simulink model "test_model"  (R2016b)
settings: Solver=VariableStepAuto  StartTime=0.0  StopTime=runtime  RelTol=1e-3
InitFcn:
  | clear mex
  | delete test_model_sfun.mexw64
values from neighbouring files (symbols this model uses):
  g = 9.81    [modelParameters.m]
  height_controlled_o = (((Rm*If        + (((omega0_o * 2 * Rm * Kv * Kq      * Kd + 1)^2) - 1)/(4* Rm*Kv^2*Kq      * Kd))/Vb)*(Pmax - Pmin) + Pmin)    [modelParameters.m]
  If = 0.3836    [modelParameters.m]
  Jreq = 4.2012e-05    [modelParameters.m]
  Jxx = 0.0130    (= 0.013)    [modelParameters.m]
  Jyy = 0.0140    (= 0.014)    [modelParameters.m]
  Jzz = 0.0285    [modelParameters.m]
  Kd = 1.4852e-07    [modelParameters.m]
  Ki_mahony = 0.001    [modelParameters.m]
  Kp_mahony = 0.4    [modelParameters.m]
  Kq = 96.3422    [modelParameters.m]
  Kt = 1.2007e-05    [modelParameters.m]
  Kv = 96.3422    [modelParameters.m]
  m = 1.216    [modelParameters.m]
  omega0_o = sqrt((m*g)/(4*Kt))    [modelParameters.m]
  omega1_o = sqrt((m*g)/(4*Kt))    [modelParameters.m]
  omega2_o = sqrt((m*g)/(4*Kt))    [modelParameters.m]
  omega3_o = sqrt((m*g)/(4*Kt))    [modelParameters.m]
  pitch_o = 0    [modelParameters.m]
  pitchrate_o = 0    [modelParameters.m]
  Pmax = 1    [modelParameters.m]
  Pmin = 0    [modelParameters.m]
  r_oc = [0; 0; 0]    [modelParameters.m]
  rhx = 0.16    [modelParameters.m]
  rhy = 0.16    [modelParameters.m]
  rhz = 0.03    [modelParameters.m]
  Rm = 0.235    [modelParameters.m]
  roll_o = 0    [modelParameters.m]
  rollrate_o = 0    [modelParameters.m]
  Tc = 0.04    [modelParameters.m]
  Tq = 0.005    [modelParameters.m]
  Vb = 11.4    [modelParameters.m]
  x_controlled_o = 0    [modelParameters.m]
  x_o = 0    [modelParameters.m]
  x_vel_o = 0    [modelParameters.m]
  y_controlled_o = 0    [modelParameters.m]
  y_o = 0    [modelParameters.m]
  y_vel_o = 0    [modelParameters.m]
  yaw_controlled_o = 0    [modelParameters.m]
  yaw_o = 0    [modelParameters.m]
  yawrate_o = 0    [modelParameters.m]
  z_o = 0    [modelParameters.m]
  z_vel_o = 0    [modelParameters.m]
undefined symbols (not defined in the file or in its folder): a, Ki, Kp, Ts
libraries: simulink x38, dsparch4 x3, vrlib x2
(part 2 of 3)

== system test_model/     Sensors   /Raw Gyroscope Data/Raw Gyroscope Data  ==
  From Workspace5 : FromWorkspace  VariableName=raw_gyro_data  SampleTime=Tq
  raw_gyro : Outport
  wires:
  From Workspace5/1 -> raw_gyro/1

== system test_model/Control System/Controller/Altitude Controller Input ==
  note: 1) Add Subsystem or Model blocks as valid variant choices. 2) You cannot connect blocks at this level. At simulation, connectivity is automatically determined, based on the active variant and port name matching.
  z_error_model : Inport
  Feedback : Subsystem  VariantControl=logAnalysisToggle==0
  z error : Subsystem  VariantControl=logAnalysisToggle==1
  z_error : Outport

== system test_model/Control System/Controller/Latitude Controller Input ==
  note: 1) Add Subsystem or Model blocks as valid variant choices. 2) You cannot connect blocks at this level. At simulation, connectivity is automatically determined, based on the active variant and port name matching.
  x_error_model : Inport
  Feedback : Subsystem  VariantControl=logAnalysisToggle==0
  x error : Subsystem  VariantControl=logAnalysisToggle==1
  x_error : Outport

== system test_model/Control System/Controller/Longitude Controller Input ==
  note: 1) Add Subsystem or Model blocks as valid variant choices. 2) You cannot connect blocks at this level. At simulation, connectivity is automatically determined, based on the active variant and port name matching.
  y_error_model : Inport
  Feedback : Subsystem  VariantControl=logAnalysisToggle==0
  y error : Subsystem  VariantControl=logAnalysisToggle==1
  y_error : Outport

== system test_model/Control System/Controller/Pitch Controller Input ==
  note: 1) Add Subsystem or Model blocks as valid variant choices. 2) You cannot connect blocks at this level. At simulation, connectivity is automatically determined, based on the active variant and port name matching.
  pitch_error_model : Inport
  Feedback : Subsystem  VariantControl=logAnalysisToggle==0
  pitch error : Subsystem  VariantControl=logAnalysisToggle==1
  pitch_error : Outport

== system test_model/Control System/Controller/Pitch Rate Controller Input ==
  note: 1) Add Subsystem or Model blocks as valid variant choices. 2) You cannot connect blocks at this level. At simulation, connectivity is automatically determined, based on the active variant and port name matching.
  pitchrate_error_model : Inport
  Feedback : Subsystem  VariantControl=logAnalysisToggle==0
  pitchrate error : Subsystem  VariantControl=logAnalysisToggle==1
  pitchrate_error : Outport

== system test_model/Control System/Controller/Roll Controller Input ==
  note: 1) Add Subsystem or Model blocks as valid variant choices. 2) You cannot connect blocks at this level. At simulation, connectivity is automatically determined, based on the active variant and port name matching.
  roll_error_model : Inport
  Feedback : Subsystem  VariantControl=logAnalysisToggle==0
  roll error : Subsystem  VariantControl=logAnalysisToggle==1
  roll_error : Outport

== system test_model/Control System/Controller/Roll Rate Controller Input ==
  note: 1) Add Subsystem or Model blocks as valid variant choices. 2) You cannot connect blocks at this level. At simulation, connectivity is automatically determined, based on the active variant and port name matching.
  rollrate_error_model : Inport
  Feedback : Subsystem  VariantControl=logAnalysisToggle==0
  rollrate error : Subsystem  VariantControl=logAnalysisToggle==1
  rollrate_error : Outport

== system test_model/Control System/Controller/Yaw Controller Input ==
  note: 1) Add Subsystem or Model blocks as valid variant choices. 2) You cannot connect blocks at this level. At simulation, connectivity is automatically determined, based on the active variant and port name matching.
  yaw_error_model : Inport
  Feedback : Subsystem  VariantControl=logAnalysisToggle==0
  yaw error : Subsystem  VariantControl=logAnalysisToggle==1
  yaw_error : Outport

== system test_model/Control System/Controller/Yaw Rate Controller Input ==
  note: 1) Add Subsystem or Model blocks as valid variant choices. 2) You cannot connect blocks at this level. At simulation, connectivity is automatically determined, based on the active variant and port name matching.
  yawrate_error_model : Inport
  Feedback : Subsystem  VariantControl=logAnalysisToggle==0
  yawrate error : Subsystem  VariantControl=logAnalysisToggle==1
  yawrate_error : Outport

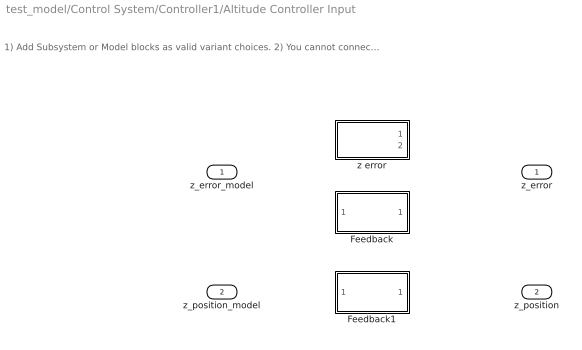
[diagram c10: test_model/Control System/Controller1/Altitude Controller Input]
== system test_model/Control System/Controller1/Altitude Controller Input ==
  note: 1) Add Subsystem or Model blocks as valid variant choices. 2) You cannot connect blocks at this level. At simulation, connectivity is automatically determined, based on the active variant and port name matching.
  z_error_model : Inport
  z_position_model : Inport  Port=2
  Feedback : Subsystem  VariantControl=logAnalysisToggle==0
  Feedback1 : Subsystem  VariantControl=logAnalysisToggle==0
  z error : Subsystem  VariantControl=logAnalysisToggle==1
  z_error : Outport
  z_position : Outport  Port=2

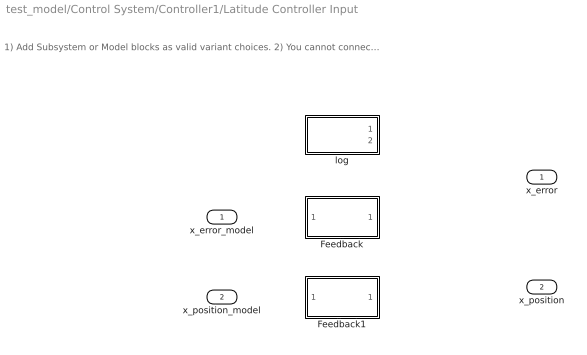
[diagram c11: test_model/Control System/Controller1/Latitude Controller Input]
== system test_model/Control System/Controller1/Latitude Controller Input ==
  note: 1) Add Subsystem or Model blocks as valid variant choices. 2) You cannot connect blocks at this level. At simulation, connectivity is automatically determined, based on the active variant and port name matching.
  x_error_model : Inport
  x_position_model : Inport  Port=2
  Feedback : Subsystem  VariantControl=logAnalysisToggle==0
  Feedback1 : Subsystem  VariantControl=logAnalysisToggle==0
  log : Subsystem  VariantControl=logAnalysisToggle==1
  x_error : Outport
  x_position : Outport  Port=2

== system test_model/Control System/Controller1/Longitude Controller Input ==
  note: 1) Add Subsystem or Model blocks as valid variant choices. 2) You cannot connect blocks at this level. At simulation, connectivity is automatically determined, based on the active variant and port name matching.
  y_error_model : Inport
  y_position_model : Inport  Port=2
  Feedback : Subsystem  VariantControl=logAnalysisToggle==0
  Feedback1 : Subsystem  VariantControl=logAnalysisToggle==0
  y error : Subsystem  VariantControl=logAnalysisToggle==1
  y_error : Outport
  y_position : Outport  Port=2

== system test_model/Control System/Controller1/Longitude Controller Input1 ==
  note: 1) Add Subsystem or Model blocks as valid variant choices. 2) You cannot connect blocks at this level. At simulation, connectivity is automatically determined, based on the active variant and port name matching.
  y_vel_error_model : Inport
  y_vel_model : Inport  Port=2
  Feedback : Subsystem  VariantControl=logAnalysisToggle==0
  Feedback1 : Subsystem  VariantControl=logAnalysisToggle==0
  y error : Subsystem  VariantControl=logAnalysisToggle==1
  y_vel_error : Outport
  y_vel : Outport  Port=2

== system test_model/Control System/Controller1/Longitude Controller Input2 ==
  note: 1) Add Subsystem or Model blocks as valid variant choices. 2) You cannot connect blocks at this level. At simulation, connectivity is automatically determined, based on the active variant and port name matching.
  x_vel_error_model : Inport
  x_vel_model : Inport  Port=2
  Feedback : Subsystem  VariantControl=logAnalysisToggle==0
  Feedback1 : Subsystem  VariantControl=logAnalysisToggle==0
  y error : Subsystem  VariantControl=logAnalysisToggle==1
  x_vel_error : Outport
  x_vel : Outport  Port=2

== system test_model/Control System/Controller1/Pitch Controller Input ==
  note: 1) Add Subsystem or Model blocks as valid variant choices. 2) You cannot connect blocks at this level. At simulation, connectivity is automatically determined, based on the active variant and port name matching.
  pitch_error_model : Inport
  pitch_angle_model : Inport  Port=2
  Feedback : Subsystem  VariantControl=logAnalysisToggle==0
  Feedback1 : Subsystem  VariantControl=logAnalysisToggle==0
  pitch error : Subsystem  VariantControl=logAnalysisToggle==1
  pitch_error : Outport
  pitch_angle : Outport  Port=2

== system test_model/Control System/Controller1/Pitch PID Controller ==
  pitch_error : Inport
  pitch_angle : Inport  Port=2
  Add : Sum  Inputs=+-
  Discrete D Controller : Subsystem  TreatAsAtomicUnit=on  SystemSampleTime=Ts
  Discrete PI Controller : simulink/Continuous/PID Controller  Controller=PI  TimeDomain=Discrete-time  SampleTime=Ts  IntegratorMethod=Forward Euler  FilterMethod=Forward Euler  Form=Parallel  UseFilter=on  ControllerParametersSource=internal  P=Kp  I=Ki  D=0  N=100  InitialConditionSource=internal  InitialConditionForIntegrator=0  InitialConditionForFilter=0  ExternalReset=none  LimitOutput=off  UpperSaturationLimit=inf  LowerSaturationLimit=-inf  LinearizeAsGain=off  AntiWindupMode=none  Kb=1  TrackingMode=off  Kt=1  PParamMin=[]  PParamMax=[]  IParamMin=[]  IParamMax=[]  DParamMin=[]  DParamMax=[]  NParamMin=[]  NParamMax=[]  KbParamMin=[]  KbParamMax=[]  KtParamMin=[]  KtParamMax=[]  POutMin=[]  POutMax=[]  IOutMin=[]  IOutMax=[]  DOutMin=[]  DOutMax=[]  NOutMin=[]  NOutMax=[]  KbOutMin=[]  KbOutMax=[]  KtOutMin=[]  KtOutMax=[]  IntegratorOutMin=[]  IntegratorOutMax=[]  FilterOutMin=[]  FilterOutMax=[]  SumOutMin=[]  SumOutMax=[]  SumI1OutMin=[]  SumI1OutMax=[]  SumI2OutMin=[]  SumI2OutMax=[]  SumI3OutMin=[]  SumI3OutMax=[]  SumDOutMin=[]  SumDOutMax=[]  SaturationOutMin=[]  SaturationOutMax=[]  IntegratorContinuousStateAttributes=''  IntegratorStateMustResolveToSignalObject=off  IntegratorRTWStateStorageClass=Auto  FilterContinuousStateAttributes=''  FilterStateMustResolveToSignalObject=off  FilterRTWStateStorageClass=Auto  DifferentiatorICPrevScaledInput=0  DifferentiatorOutMin=[]  DifferentiatorOutMax=[]
  pitchrate_setpoint : Outport
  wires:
  pitch_angle/1 -> Discrete D Controller/1(pitch_angle)
  pitch_error/1 -> Discrete PI Controller/1
  Discrete PI Controller/1 -> Add/1
  Discrete D Controller/1(output) -> Add/2
  Add/1 -> pitchrate_setpoint/1

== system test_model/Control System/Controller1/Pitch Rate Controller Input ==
  note: 1) Add Subsystem or Model blocks as valid variant choices. 2) You cannot connect blocks at this level. At simulation, connectivity is automatically determined, based on the active variant and port name matching.
  pitchrate_error_model : Inport
  pitchrate_model : Inport  Port=2
  Feedback : Subsystem  VariantControl=logAnalysisToggle==0
  Feedback1 : Subsystem  VariantControl=logAnalysisToggle==0
  pitchrate error : Subsystem  VariantControl=logAnalysisToggle==1
  pitchrate_error : Outport
  pitchrate : Outport  Port=2

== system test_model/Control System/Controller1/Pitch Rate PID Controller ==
  pitchrate_error : Inport
  pitchrate : Inport  Port=2
  Add : Sum  Inputs=+-
  Discrete D Controller : Subsystem  TreatAsAtomicUnit=on  SystemSampleTime=Ts
  Discrete PI Controller : simulink/Continuous/PID Controller  Controller=PI  TimeDomain=Discrete-time  SampleTime=Ts  IntegratorMethod=Forward Euler  FilterMethod=Forward Euler  Form=Parallel  UseFilter=on  ControllerParametersSource=internal  P=Kp  I=Ki  D=0  N=100  InitialConditionSource=internal  InitialConditionForIntegrator=0  InitialConditionForFilter=0  ExternalReset=none  LimitOutput=off  UpperSaturationLimit=inf  LowerSaturationLimit=-inf  LinearizeAsGain=off  AntiWindupMode=none  Kb=1  TrackingMode=off  Kt=1  PParamMin=[]  PParamMax=[]  IParamMin=[]  IParamMax=[]  DParamMin=[]  DParamMax=[]  NParamMin=[]  NParamMax=[]  KbParamMin=[]  KbParamMax=[]  KtParamMin=[]  KtParamMax=[]  POutMin=[]  POutMax=[]  IOutMin=[]  IOutMax=[]  DOutMin=[]  DOutMax=[]  NOutMin=[]  NOutMax=[]  KbOutMin=[]  KbOutMax=[]  KtOutMin=[]  KtOutMax=[]  IntegratorOutMin=[]  IntegratorOutMax=[]  FilterOutMin=[]  FilterOutMax=[]  SumOutMin=[]  SumOutMax=[]  SumI1OutMin=[]  SumI1OutMax=[]  SumI2OutMin=[]  SumI2OutMax=[]  SumI3OutMin=[]  SumI3OutMax=[]  SumDOutMin=[]  SumDOutMax=[]  SaturationOutMin=[]  SaturationOutMax=[]  IntegratorContinuousStateAttributes=''  IntegratorStateMustResolveToSignalObject=off  IntegratorRTWStateStorageClass=Auto  FilterContinuousStateAttributes=''  FilterStateMustResolveToSignalObject=off  FilterRTWStateStorageClass=Auto  DifferentiatorICPrevScaledInput=0  DifferentiatorOutMin=[]  DifferentiatorOutMax=[]
  x_motor_command : Outport
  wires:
  pitchrate/1 -> Discrete D Controller/1(pitch_angle)
  pitchrate_error/1 -> Discrete PI Controller/1
  Discrete PI Controller/1 -> Add/1
  Discrete D Controller/1(output) -> Add/2
  Add/1 -> x_motor_command/1

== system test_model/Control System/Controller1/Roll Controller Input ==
  note: 1) Add Subsystem or Model blocks as valid variant choices. 2) You cannot connect blocks at this level. At simulation, connectivity is automatically determined, based on the active variant and port name matching.
  roll_error_model : Inport
  roll_angle_model : Inport  Port=2
  Feedback : Subsystem  VariantControl=logAnalysisToggle==0
  Feedback1 : Subsystem  VariantControl=logAnalysisToggle==0
  roll error : Subsystem  VariantControl=logAnalysisToggle==1
  roll_error : Outport
  roll_angle : Outport  Port=2

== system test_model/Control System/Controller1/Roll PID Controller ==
  roll_error : Inport
  roll_angle : Inport  Port=2
  Add : Sum  Inputs=+-
  Discrete D Controller : Subsystem  TreatAsAtomicUnit=on  SystemSampleTime=Ts
  Discrete PI Controller : simulink/Continuous/PID Controller  Controller=PI  TimeDomain=Discrete-time  SampleTime=Ts  IntegratorMethod=Forward Euler  FilterMethod=Forward Euler  Form=Parallel  UseFilter=on  ControllerParametersSource=internal  P=Kp  I=Ki  D=0  N=100  InitialConditionSource=internal  InitialConditionForIntegrator=0  InitialConditionForFilter=0  ExternalReset=none  LimitOutput=off  UpperSaturationLimit=inf  LowerSaturationLimit=-inf  LinearizeAsGain=off  AntiWindupMode=none  Kb=1  TrackingMode=off  Kt=1  PParamMin=[]  PParamMax=[]  IParamMin=[]  IParamMax=[]  DParamMin=[]  DParamMax=[]  NParamMin=[]  NParamMax=[]  KbParamMin=[]  KbParamMax=[]  KtParamMin=[]  KtParamMax=[]  POutMin=[]  POutMax=[]  IOutMin=[]  IOutMax=[]  DOutMin=[]  DOutMax=[]  NOutMin=[]  NOutMax=[]  KbOutMin=[]  KbOutMax=[]  KtOutMin=[]  KtOutMax=[]  IntegratorOutMin=[]  IntegratorOutMax=[]  FilterOutMin=[]  FilterOutMax=[]  SumOutMin=[]  SumOutMax=[]  SumI1OutMin=[]  SumI1OutMax=[]  SumI2OutMin=[]  SumI2OutMax=[]  SumI3OutMin=[]  SumI3OutMax=[]  SumDOutMin=[]  SumDOutMax=[]  SaturationOutMin=[]  SaturationOutMax=[]  IntegratorContinuousStateAttributes=''  IntegratorStateMustResolveToSignalObject=off  IntegratorRTWStateStorageClass=Auto  FilterContinuousStateAttributes=''  FilterStateMustResolveToSignalObject=off  FilterRTWStateStorageClass=Auto  DifferentiatorICPrevScaledInput=0  DifferentiatorOutMin=[]  DifferentiatorOutMax=[]
  rollrate_setpoint : Outport
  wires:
  roll_angle/1 -> Discrete D Controller/1(pitch_angle)
  roll_error/1 -> Discrete PI Controller/1
  Discrete PI Controller/1 -> Add/1
  Discrete D Controller/1(output) -> Add/2
  Add/1 -> rollrate_setpoint/1

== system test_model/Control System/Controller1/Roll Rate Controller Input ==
  note: 1) Add Subsystem or Model blocks as valid variant choices. 2) You cannot connect blocks at this level. At simulation, connectivity is automatically determined, based on the active variant and port name matching.
  rollrate_error_model : Inport
  rollrate_model : Inport  Port=2
  Feedback : Subsystem  VariantControl=logAnalysisToggle==0
  Feedback1 : Subsystem  VariantControl=logAnalysisToggle==0
  rollrate error : Subsystem  VariantControl=logAnalysisToggle==1
  rollrate_error : Outport
  rollrate : Outport  Port=2

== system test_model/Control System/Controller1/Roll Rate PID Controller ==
  rollrate_error : Inport
  rollrate : Inport  Port=2
  Add : Sum  Inputs=+-
  Discrete D Controller : Subsystem  TreatAsAtomicUnit=on  SystemSampleTime=Ts
  Discrete PI Controller : simulink/Continuous/PID Controller  Controller=PI  TimeDomain=Discrete-time  SampleTime=Ts  IntegratorMethod=Forward Euler  FilterMethod=Forward Euler  Form=Parallel  UseFilter=on  ControllerParametersSource=internal  P=Kp  I=Ki  D=0  N=100  InitialConditionSource=internal  InitialConditionForIntegrator=0  InitialConditionForFilter=0  ExternalReset=none  LimitOutput=off  UpperSaturationLimit=inf  LowerSaturationLimit=-inf  LinearizeAsGain=off  AntiWindupMode=none  Kb=1  TrackingMode=off  Kt=1  PParamMin=[]  PParamMax=[]  IParamMin=[]  IParamMax=[]  DParamMin=[]  DParamMax=[]  NParamMin=[]  NParamMax=[]  KbParamMin=[]  KbParamMax=[]  KtParamMin=[]  KtParamMax=[]  POutMin=[]  POutMax=[]  IOutMin=[]  IOutMax=[]  DOutMin=[]  DOutMax=[]  NOutMin=[]  NOutMax=[]  KbOutMin=[]  KbOutMax=[]  KtOutMin=[]  KtOutMax=[]  IntegratorOutMin=[]  IntegratorOutMax=[]  FilterOutMin=[]  FilterOutMax=[]  SumOutMin=[]  SumOutMax=[]  SumI1OutMin=[]  SumI1OutMax=[]  SumI2OutMin=[]  SumI2OutMax=[]  SumI3OutMin=[]  SumI3OutMax=[]  SumDOutMin=[]  SumDOutMax=[]  SaturationOutMin=[]  SaturationOutMax=[]  IntegratorContinuousStateAttributes=''  IntegratorStateMustResolveToSignalObject=off  IntegratorRTWStateStorageClass=Auto  FilterContinuousStateAttributes=''  FilterStateMustResolveToSignalObject=off  FilterRTWStateStorageClass=Auto  DifferentiatorICPrevScaledInput=0  DifferentiatorOutMin=[]  DifferentiatorOutMax=[]
  y_motor_command : Outport
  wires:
  rollrate/1 -> Discrete D Controller/1(pitch_angle)
  rollrate_error/1 -> Discrete PI Controller/1
  Discrete PI Controller/1 -> Add/1
  Discrete D Controller/1(output) -> Add/2
  Add/1 -> y_motor_command/1

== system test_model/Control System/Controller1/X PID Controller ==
  x_error : Inport
  x_pos : Inport  Port=2
  Add : Sum  Inputs=+-
  Discrete D Controller : Subsystem  TreatAsAtomicUnit=on  SystemSampleTime=Ts
  Discrete PI Controller : simulink/Continuous/PID Controller  Controller=PI  TimeDomain=Discrete-time  SampleTime=Ts  IntegratorMethod=Forward Euler  FilterMethod=Forward Euler  Form=Parallel  UseFilter=on  ControllerParametersSource=internal  P=Kp  I=Ki  D=0  N=100  InitialConditionSource=internal  InitialConditionForIntegrator=0  InitialConditionForFilter=0  ExternalReset=none  LimitOutput=off  UpperSaturationLimit=inf  LowerSaturationLimit=-inf  LinearizeAsGain=off  AntiWindupMode=none  Kb=1  TrackingMode=off  Kt=1  PParamMin=[]  PParamMax=[]  IParamMin=[]  IParamMax=[]  DParamMin=[]  DParamMax=[]  NParamMin=[]  NParamMax=[]  KbParamMin=[]  KbParamMax=[]  KtParamMin=[]  KtParamMax=[]  POutMin=[]  POutMax=[]  IOutMin=[]  IOutMax=[]  DOutMin=[]  DOutMax=[]  NOutMin=[]  NOutMax=[]  KbOutMin=[]  KbOutMax=[]  KtOutMin=[]  KtOutMax=[]  IntegratorOutMin=[]  IntegratorOutMax=[]  FilterOutMin=[]  FilterOutMax=[]  SumOutMin=[]  SumOutMax=[]  SumI1OutMin=[]  SumI1OutMax=[]  SumI2OutMin=[]  SumI2OutMax=[]  SumI3OutMin=[]  SumI3OutMax=[]  SumDOutMin=[]  SumDOutMax=[]  SaturationOutMin=[]  SaturationOutMax=[]  IntegratorContinuousStateAttributes=''  IntegratorStateMustResolveToSignalObject=off  IntegratorRTWStateStorageClass=Auto  FilterContinuousStateAttributes=''  FilterStateMustResolveToSignalObject=off  FilterRTWStateStorageClass=Auto  DifferentiatorICPrevScaledInput=0  DifferentiatorOutMin=[]  DifferentiatorOutMax=[]
  pitch_setpoint : Outport
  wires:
  x_pos/1 -> Discrete D Controller/1(x_pos)
  x_error/1 -> Discrete PI Controller/1
  Discrete PI Controller/1 -> Add/1
  Discrete D Controller/1(output) -> Add/2
  Add/1 -> pitch_setpoint/1

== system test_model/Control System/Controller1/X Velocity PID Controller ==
  x_vel_error : Inport
  x_vel : Inport  Port=2
  Add : Sum  Inputs=+-
  Discrete D Controller : Subsystem  TreatAsAtomicUnit=on  SystemSampleTime=Ts
  Discrete PI Controller : simulink/Continuous/PID Controller  Controller=PI  TimeDomain=Discrete-time  SampleTime=Ts  IntegratorMethod=Forward Euler  FilterMethod=Forward Euler  Form=Parallel  UseFilter=on  ControllerParametersSource=internal  P=Kp  I=Ki  D=0  N=100  InitialConditionSource=internal  InitialConditionForIntegrator=0  InitialConditionForFilter=0  ExternalReset=none  LimitOutput=off  UpperSaturationLimit=inf  LowerSaturationLimit=-inf  LinearizeAsGain=off  AntiWindupMode=none  Kb=1  TrackingMode=off  Kt=1  PParamMin=[]  PParamMax=[]  IParamMin=[]  IParamMax=[]  DParamMin=[]  DParamMax=[]  NParamMin=[]  NParamMax=[]  KbParamMin=[]  KbParamMax=[]  KtParamMin=[]  KtParamMax=[]  POutMin=[]  POutMax=[]  IOutMin=[]  IOutMax=[]  DOutMin=[]  DOutMax=[]  NOutMin=[]  NOutMax=[]  KbOutMin=[]  KbOutMax=[]  KtOutMin=[]  KtOutMax=[]  IntegratorOutMin=[]  IntegratorOutMax=[]  FilterOutMin=[]  FilterOutMax=[]  SumOutMin=[]  SumOutMax=[]  SumI1OutMin=[]  SumI1OutMax=[]  SumI2OutMin=[]  SumI2OutMax=[]  SumI3OutMin=[]  SumI3OutMax=[]  SumDOutMin=[]  SumDOutMax=[]  SaturationOutMin=[]  SaturationOutMax=[]  IntegratorContinuousStateAttributes=''  IntegratorStateMustResolveToSignalObject=off  IntegratorRTWStateStorageClass=Auto  FilterContinuousStateAttributes=''  FilterStateMustResolveToSignalObject=off  FilterRTWStateStorageClass=Auto  DifferentiatorICPrevScaledInput=0  DifferentiatorOutMin=[]  DifferentiatorOutMax=[]
  pitch_setpoint : Outport
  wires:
  x_vel/1 -> Discrete D Controller/1(x_vel)
  x_vel_error/1 -> Discrete PI Controller/1
  Discrete PI Controller/1 -> Add/1
  Discrete D Controller/1(output) -> Add/2
  Add/1 -> pitch_setpoint/1

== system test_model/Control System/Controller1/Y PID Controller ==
  y_error : Inport
  y_pos : Inport  Port=2
  Add : Sum  Inputs=+-
  Discrete D Controller : Subsystem  TreatAsAtomicUnit=on  SystemSampleTime=Ts
  Discrete PI Controller : simulink/Continuous/PID Controller  Controller=PI  TimeDomain=Discrete-time  SampleTime=Ts  IntegratorMethod=Forward Euler  FilterMethod=Forward Euler  Form=Parallel  UseFilter=on  ControllerParametersSource=internal  P=Kp  I=Ki  D=0  N=100  InitialConditionSource=internal  InitialConditionForIntegrator=0  InitialConditionForFilter=0  ExternalReset=none  LimitOutput=off  UpperSaturationLimit=inf  LowerSaturationLimit=-inf  LinearizeAsGain=off  AntiWindupMode=none  Kb=1  TrackingMode=off  Kt=1  PParamMin=[]  PParamMax=[]  IParamMin=[]  IParamMax=[]  DParamMin=[]  DParamMax=[]  NParamMin=[]  NParamMax=[]  KbParamMin=[]  KbParamMax=[]  KtParamMin=[]  KtParamMax=[]  POutMin=[]  POutMax=[]  IOutMin=[]  IOutMax=[]  DOutMin=[]  DOutMax=[]  NOutMin=[]  NOutMax=[]  KbOutMin=[]  KbOutMax=[]  KtOutMin=[]  KtOutMax=[]  IntegratorOutMin=[]  IntegratorOutMax=[]  FilterOutMin=[]  FilterOutMax=[]  SumOutMin=[]  SumOutMax=[]  SumI1OutMin=[]  SumI1OutMax=[]  SumI2OutMin=[]  SumI2OutMax=[]  SumI3OutMin=[]  SumI3OutMax=[]  SumDOutMin=[]  SumDOutMax=[]  SaturationOutMin=[]  SaturationOutMax=[]  IntegratorContinuousStateAttributes=''  IntegratorStateMustResolveToSignalObject=off  IntegratorRTWStateStorageClass=Auto  FilterContinuousStateAttributes=''  FilterStateMustResolveToSignalObject=off  FilterRTWStateStorageClass=Auto  DifferentiatorICPrevScaledInput=0  DifferentiatorOutMin=[]  DifferentiatorOutMax=[]
  roll_setpoint : Outport
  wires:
  y_pos/1 -> Discrete D Controller/1(y_pos)
  y_error/1 -> Discrete PI Controller/1
  Discrete PI Controller/1 -> Add/1
  Discrete D Controller/1(output) -> Add/2
  Add/1 -> roll_setpoint/1

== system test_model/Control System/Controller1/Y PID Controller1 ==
  y_error : Inport
  y_pos : Inport  Port=2
  Add : Sum  Inputs=+-
  Discrete D Controller : Subsystem  TreatAsAtomicUnit=on  SystemSampleTime=Ts
  Discrete PI Controller : simulink/Continuous/PID Controller  Controller=PI  TimeDomain=Discrete-time  SampleTime=Ts  IntegratorMethod=Forward Euler  FilterMethod=Forward Euler  Form=Parallel  UseFilter=on  ControllerParametersSource=internal  P=Kp  I=Ki  D=0  N=100  InitialConditionSource=internal  InitialConditionForIntegrator=0  InitialConditionForFilter=0  ExternalReset=none  LimitOutput=off  UpperSaturationLimit=inf  LowerSaturationLimit=-inf  LinearizeAsGain=off  AntiWindupMode=none  Kb=1  TrackingMode=off  Kt=1  PParamMin=[]  PParamMax=[]  IParamMin=[]  IParamMax=[]  DParamMin=[]  DParamMax=[]  NParamMin=[]  NParamMax=[]  KbParamMin=[]  KbParamMax=[]  KtParamMin=[]  KtParamMax=[]  POutMin=[]  POutMax=[]  IOutMin=[]  IOutMax=[]  DOutMin=[]  DOutMax=[]  NOutMin=[]  NOutMax=[]  KbOutMin=[]  KbOutMax=[]  KtOutMin=[]  KtOutMax=[]  IntegratorOutMin=[]  IntegratorOutMax=[]  FilterOutMin=[]  FilterOutMax=[]  SumOutMin=[]  SumOutMax=[]  SumI1OutMin=[]  SumI1OutMax=[]  SumI2OutMin=[]  SumI2OutMax=[]  SumI3OutMin=[]  SumI3OutMax=[]  SumDOutMin=[]  SumDOutMax=[]  SaturationOutMin=[]  SaturationOutMax=[]  IntegratorContinuousStateAttributes=''  IntegratorStateMustResolveToSignalObject=off  IntegratorRTWStateStorageClass=Auto  FilterContinuousStateAttributes=''  FilterStateMustResolveToSignalObject=off  FilterRTWStateStorageClass=Auto  DifferentiatorICPrevScaledInput=0  DifferentiatorOutMin=[]  DifferentiatorOutMax=[]
  y_vel_setpoint : Outport
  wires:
  y_pos/1 -> Discrete D Controller/1(y_pos)
  y_error/1 -> Discrete PI Controller/1
  Discrete PI Controller/1 -> Add/1
  Discrete D Controller/1(output) -> Add/2
  Add/1 -> y_vel_setpoint/1

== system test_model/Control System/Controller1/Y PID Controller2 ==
  x_error : Inport
  x_pos : Inport  Port=2
  Add : Sum  Inputs=+-
  Discrete D Controller : Subsystem  TreatAsAtomicUnit=on  SystemSampleTime=Ts
  Discrete PI Controller : simulink/Continuous/PID Controller  Controller=PI  TimeDomain=Discrete-time  SampleTime=Ts  IntegratorMethod=Forward Euler  FilterMethod=Forward Euler  Form=Parallel  UseFilter=on  ControllerParametersSource=internal  P=Kp  I=Ki  D=0  N=100  InitialConditionSource=internal  InitialConditionForIntegrator=0  InitialConditionForFilter=0  ExternalReset=none  LimitOutput=off  UpperSaturationLimit=inf  LowerSaturationLimit=-inf  LinearizeAsGain=off  AntiWindupMode=none  Kb=1  TrackingMode=off  Kt=1  PParamMin=[]  PParamMax=[]  IParamMin=[]  IParamMax=[]  DParamMin=[]  DParamMax=[]  NParamMin=[]  NParamMax=[]  KbParamMin=[]  KbParamMax=[]  KtParamMin=[]  KtParamMax=[]  POutMin=[]  POutMax=[]  IOutMin=[]  IOutMax=[]  DOutMin=[]  DOutMax=[]  NOutMin=[]  NOutMax=[]  KbOutMin=[]  KbOutMax=[]  KtOutMin=[]  KtOutMax=[]  IntegratorOutMin=[]  IntegratorOutMax=[]  FilterOutMin=[]  FilterOutMax=[]  SumOutMin=[]  SumOutMax=[]  SumI1OutMin=[]  SumI1OutMax=[]  SumI2OutMin=[]  SumI2OutMax=[]  SumI3OutMin=[]  SumI3OutMax=[]  SumDOutMin=[]  SumDOutMax=[]  SaturationOutMin=[]  SaturationOutMax=[]  IntegratorContinuousStateAttributes=''  IntegratorStateMustResolveToSignalObject=off  IntegratorRTWStateStorageClass=Auto  FilterContinuousStateAttributes=''  FilterStateMustResolveToSignalObject=off  FilterRTWStateStorageClass=Auto  DifferentiatorICPrevScaledInput=0  DifferentiatorOutMin=[]  DifferentiatorOutMax=[]
  x_vel_setpoint : Outport
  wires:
  x_pos/1 -> Discrete D Controller/1(x_pos)
  x_error/1 -> Discrete PI Controller/1
  Discrete PI Controller/1 -> Add/1
  Discrete D Controller/1(output) -> Add/2
  Add/1 -> x_vel_setpoint/1

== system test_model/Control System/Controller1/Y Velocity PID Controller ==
  y_error : Inport
  y_pos : Inport  Port=2
  Add : Sum  Inputs=+-
  Discrete D Controller : Subsystem  TreatAsAtomicUnit=on  SystemSampleTime=Ts
  Discrete PI Controller : simulink/Continuous/PID Controller  Controller=PI  TimeDomain=Discrete-time  SampleTime=Ts  IntegratorMethod=Forward Euler  FilterMethod=Forward Euler  Form=Parallel  UseFilter=on  ControllerParametersSource=internal  P=Kp  I=Ki  D=0  N=100  InitialConditionSource=internal  InitialConditionForIntegrator=0  InitialConditionForFilter=0  ExternalReset=none  LimitOutput=off  UpperSaturationLimit=inf  LowerSaturationLimit=-inf  LinearizeAsGain=off  AntiWindupMode=none  Kb=1  TrackingMode=off  Kt=1  PParamMin=[]  PParamMax=[]  IParamMin=[]  IParamMax=[]  DParamMin=[]  DParamMax=[]  NParamMin=[]  NParamMax=[]  KbParamMin=[]  KbParamMax=[]  KtParamMin=[]  KtParamMax=[]  POutMin=[]  POutMax=[]  IOutMin=[]  IOutMax=[]  DOutMin=[]  DOutMax=[]  NOutMin=[]  NOutMax=[]  KbOutMin=[]  KbOutMax=[]  KtOutMin=[]  KtOutMax=[]  IntegratorOutMin=[]  IntegratorOutMax=[]  FilterOutMin=[]  FilterOutMax=[]  SumOutMin=[]  SumOutMax=[]  SumI1OutMin=[]  SumI1OutMax=[]  SumI2OutMin=[]  SumI2OutMax=[]  SumI3OutMin=[]  SumI3OutMax=[]  SumDOutMin=[]  SumDOutMax=[]  SaturationOutMin=[]  SaturationOutMax=[]  IntegratorContinuousStateAttributes=''  IntegratorStateMustResolveToSignalObject=off  IntegratorRTWStateStorageClass=Auto  FilterContinuousStateAttributes=''  FilterStateMustResolveToSignalObject=off  FilterRTWStateStorageClass=Auto  DifferentiatorICPrevScaledInput=0  DifferentiatorOutMin=[]  DifferentiatorOutMax=[]
  roll_setpoint : Outport
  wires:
  y_pos/1 -> Discrete D Controller/1(y_pos)
  y_error/1 -> Discrete PI Controller/1
  Discrete PI Controller/1 -> Add/1
  Discrete D Controller/1(output) -> Add/2
  Add/1 -> roll_setpoint/1

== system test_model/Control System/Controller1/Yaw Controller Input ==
  note: 1) Add Subsystem or Model blocks as valid variant choices. 2) You cannot connect blocks at this level. At simulation, connectivity is automatically determined, based on the active variant and port name matching.
  yaw_error_model : Inport
  yaw_angle_model : Inport  Port=2
  Feedback : Subsystem  VariantControl=logAnalysisToggle==0
  Feedback1 : Subsystem  VariantControl=logAnalysisToggle==0
  yaw error : Subsystem  VariantControl=logAnalysisToggle==1
  yaw_error : Outport
  yaw_angle : Outport  Port=2

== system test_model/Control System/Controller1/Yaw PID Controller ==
  yaw_error : Inport
  yaw_angle : Inport  Port=2
  Add : Sum  Inputs=+-
  Discrete D Controller : Subsystem  TreatAsAtomicUnit=on  SystemSampleTime=Ts
  Discrete PI Controller : simulink/Continuous/PID Controller  Controller=PI  TimeDomain=Discrete-time  SampleTime=Ts  IntegratorMethod=Forward Euler  FilterMethod=Forward Euler  Form=Parallel  UseFilter=on  ControllerParametersSource=internal  P=Kp  I=Ki  D=0  N=100  InitialConditionSource=internal  InitialConditionForIntegrator=0  InitialConditionForFilter=0  ExternalReset=none  LimitOutput=off  UpperSaturationLimit=inf  LowerSaturationLimit=-inf  LinearizeAsGain=off  AntiWindupMode=none  Kb=1  TrackingMode=off  Kt=1  PParamMin=[]  PParamMax=[]  IParamMin=[]  IParamMax=[]  DParamMin=[]  DParamMax=[]  NParamMin=[]  NParamMax=[]  KbParamMin=[]  KbParamMax=[]  KtParamMin=[]  KtParamMax=[]  POutMin=[]  POutMax=[]  IOutMin=[]  IOutMax=[]  DOutMin=[]  DOutMax=[]  NOutMin=[]  NOutMax=[]  KbOutMin=[]  KbOutMax=[]  KtOutMin=[]  KtOutMax=[]  IntegratorOutMin=[]  IntegratorOutMax=[]  FilterOutMin=[]  FilterOutMax=[]  SumOutMin=[]  SumOutMax=[]  SumI1OutMin=[]  SumI1OutMax=[]  SumI2OutMin=[]  SumI2OutMax=[]  SumI3OutMin=[]  SumI3OutMax=[]  SumDOutMin=[]  SumDOutMax=[]  SaturationOutMin=[]  SaturationOutMax=[]  IntegratorContinuousStateAttributes=''  IntegratorStateMustResolveToSignalObject=off  IntegratorRTWStateStorageClass=Auto  FilterContinuousStateAttributes=''  FilterStateMustResolveToSignalObject=off  FilterRTWStateStorageClass=Auto  DifferentiatorICPrevScaledInput=0  DifferentiatorOutMin=[]  DifferentiatorOutMax=[]
  yawrate_setpoint : Outport
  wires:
  yaw_angle/1 -> Discrete D Controller/1(yaw_pos)
  yaw_error/1 -> Discrete PI Controller/1
  Discrete PI Controller/1 -> Add/1
  Discrete D Controller/1(output) -> Add/2
  Add/1 -> yawrate_setpoint/1

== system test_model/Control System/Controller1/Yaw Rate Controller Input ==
  note: 1) Add Subsystem or Model blocks as valid variant choices. 2) You cannot connect blocks at this level. At simulation, connectivity is automatically determined, based on the active variant and port name matching.
  yawrate_error_model : Inport
  yawrate_model : Inport  Port=2
  Feedback : Subsystem  VariantControl=logAnalysisToggle==0
  Feedback1 : Subsystem  VariantControl=logAnalysisToggle==0
  yawrate error : Subsystem  VariantControl=logAnalysisToggle==1
  yawrate_error : Outport
  yawrate : Outport  Port=2

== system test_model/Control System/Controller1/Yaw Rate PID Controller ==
  yawrate_error : Inport
  yawrate : Inport  Port=2
  Add : Sum  Inputs=+-
  Discrete D Controller : Subsystem  TreatAsAtomicUnit=on  SystemSampleTime=Ts
  Discrete PI Controller : simulink/Continuous/PID Controller  Controller=PI  TimeDomain=Discrete-time  SampleTime=Ts  IntegratorMethod=Forward Euler  FilterMethod=Forward Euler  Form=Parallel  UseFilter=on  ControllerParametersSource=internal  P=Kp  I=Ki  D=0  N=100  InitialConditionSource=internal  InitialConditionForIntegrator=0  InitialConditionForFilter=0  ExternalReset=none  LimitOutput=off  UpperSaturationLimit=inf  LowerSaturationLimit=-inf  LinearizeAsGain=off  AntiWindupMode=none  Kb=1  TrackingMode=off  Kt=1  PParamMin=[]  PParamMax=[]  IParamMin=[]  IParamMax=[]  DParamMin=[]  DParamMax=[]  NParamMin=[]  NParamMax=[]  KbParamMin=[]  KbParamMax=[]  KtParamMin=[]  KtParamMax=[]  POutMin=[]  POutMax=[]  IOutMin=[]  IOutMax=[]  DOutMin=[]  DOutMax=[]  NOutMin=[]  NOutMax=[]  KbOutMin=[]  KbOutMax=[]  KtOutMin=[]  KtOutMax=[]  IntegratorOutMin=[]  IntegratorOutMax=[]  FilterOutMin=[]  FilterOutMax=[]  SumOutMin=[]  SumOutMax=[]  SumI1OutMin=[]  SumI1OutMax=[]  SumI2OutMin=[]  SumI2OutMax=[]  SumI3OutMin=[]  SumI3OutMax=[]  SumDOutMin=[]  SumDOutMax=[]  SaturationOutMin=[]  SaturationOutMax=[]  IntegratorContinuousStateAttributes=''  IntegratorStateMustResolveToSignalObject=off  IntegratorRTWStateStorageClass=Auto  FilterContinuousStateAttributes=''  FilterStateMustResolveToSignalObject=off  FilterRTWStateStorageClass=Auto  DifferentiatorICPrevScaledInput=0  DifferentiatorOutMin=[]  DifferentiatorOutMax=[]
  yaw_motor_command : Outport
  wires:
  yawrate/1 -> Discrete D Controller/1(yawrate)
  yawrate_error/1 -> Discrete PI Controller/1
  Discrete PI Controller/1 -> Add/1
  Discrete D Controller/1(output) -> Add/2
  Add/1 -> yaw_motor_command/1

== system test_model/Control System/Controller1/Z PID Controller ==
  z_error : Inport
  z_pos : Inport  Port=2
  Add : Sum  Inputs=+-
  Discrete D Controller : Subsystem  TreatAsAtomicUnit=on  SystemSampleTime=Ts
  Discrete PI Controller : simulink/Continuous/PID Controller  Controller=PI  TimeDomain=Discrete-time  SampleTime=Ts  IntegratorMethod=Forward Euler  FilterMethod=Forward Euler  Form=Parallel  UseFilter=on  ControllerParametersSource=internal  P=Kp  I=Ki  D=0  N=100  InitialConditionSource=internal  InitialConditionForIntegrator=0  InitialConditionForFilter=0  ExternalReset=none  LimitOutput=off  UpperSaturationLimit=inf  LowerSaturationLimit=-inf  LinearizeAsGain=off  AntiWindupMode=none  Kb=1  TrackingMode=off  Kt=1  PParamMin=[]  PParamMax=[]  IParamMin=[]  IParamMax=[]  DParamMin=[]  DParamMax=[]  NParamMin=[]  NParamMax=[]  KbParamMin=[]  KbParamMax=[]  KtParamMin=[]  KtParamMax=[]  POutMin=[]  POutMax=[]  IOutMin=[]  IOutMax=[]  DOutMin=[]  DOutMax=[]  NOutMin=[]  NOutMax=[]  KbOutMin=[]  KbOutMax=[]  KtOutMin=[]  KtOutMax=[]  IntegratorOutMin=[]  IntegratorOutMax=[]  FilterOutMin=[]  FilterOutMax=[]  SumOutMin=[]  SumOutMax=[]  SumI1OutMin=[]  SumI1OutMax=[]  SumI2OutMin=[]  SumI2OutMax=[]  SumI3OutMin=[]  SumI3OutMax=[]  SumDOutMin=[]  SumDOutMax=[]  SaturationOutMin=[]  SaturationOutMax=[]  IntegratorContinuousStateAttributes=''  IntegratorStateMustResolveToSignalObject=off  IntegratorRTWStateStorageClass=Auto  FilterContinuousStateAttributes=''  FilterStateMustResolveToSignalObject=off  FilterRTWStateStorageClass=Auto  DifferentiatorICPrevScaledInput=0  DifferentiatorOutMin=[]  DifferentiatorOutMax=[]
  z_motor_command : Outport
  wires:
  z_pos/1 -> Discrete D Controller/1(z_pos)
  z_error/1 -> Discrete PI Controller/1
  Discrete PI Controller/1 -> Add/1
  Discrete D Controller/1(output) -> Add/2
  Add/1 -> z_motor_command/1

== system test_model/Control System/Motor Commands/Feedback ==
  z_command_model : Inport
  z_command : Outport
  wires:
  z_command_model/1 -> z_command/1

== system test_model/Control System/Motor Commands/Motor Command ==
  From Workspace5 : FromWorkspace  VariableName=motor_commands  SampleTime=Tq
  z_command : Outport
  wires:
  From Workspace5/1 -> z_command/1

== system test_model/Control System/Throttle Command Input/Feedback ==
  z_command_model : Inport
  z_command : Outport
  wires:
  z_command_model/1 -> z_command/1

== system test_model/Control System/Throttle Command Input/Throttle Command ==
  From Workspace5 : FromWorkspace  VariableName=throttle_command  SampleTime=Tq
  z_command : Outport
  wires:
  From Workspace5/1 -> z_command/1

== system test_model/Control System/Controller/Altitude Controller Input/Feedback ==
  z_error_model : Inport
  z_error : Outport
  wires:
  z_error_model/1 -> z_error/1

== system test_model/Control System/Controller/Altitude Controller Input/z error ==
  From Workspace6 : FromWorkspace  VariableName=z_error  SampleTime=Tc  Interpolate=off  OutputAfterFinalValue=Holding final value
  z_error : Outport
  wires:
  From Workspace6/1 -> z_error/1

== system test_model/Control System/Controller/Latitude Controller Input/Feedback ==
  x_error_model : Inport
  x_error : Outport
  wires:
  x_error_model/1 -> x_error/1

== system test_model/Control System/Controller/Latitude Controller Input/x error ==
  From Workspace : FromWorkspace  VariableName=x_error  SampleTime=Tc  Interpolate=off  OutputAfterFinalValue=Holding final value
  x_error : Outport
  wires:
  From Workspace/1 -> x_error/1

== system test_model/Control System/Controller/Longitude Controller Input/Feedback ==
  y_error_model : Inport
  y_error : Outport
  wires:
  y_error_model/1 -> y_error/1

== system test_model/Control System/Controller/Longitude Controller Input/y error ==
  From Workspace3 : FromWorkspace  VariableName=y_error  SampleTime=Tc  Interpolate=off  OutputAfterFinalValue=Holding final value
  y_error : Outport
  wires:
  From Workspace3/1 -> y_error/1

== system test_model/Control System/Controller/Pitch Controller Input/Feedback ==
  pitch_error_model : Inport
  pitch_error : Outport
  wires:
  pitch_error_model/1 -> pitch_error/1

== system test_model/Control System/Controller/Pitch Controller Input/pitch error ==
  From Workspace : FromWorkspace  VariableName=pitch_error  SampleTime=Tq  Interpolate=off  OutputAfterFinalValue=Holding final value
  pitch_error : Outport
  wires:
  From Workspace/1 -> pitch_error/1

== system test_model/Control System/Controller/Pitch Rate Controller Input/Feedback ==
  pitchrate_error_model : Inport
  pitchrate_error : Outport
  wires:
  pitchrate_error_model/1 -> pitchrate_error/1

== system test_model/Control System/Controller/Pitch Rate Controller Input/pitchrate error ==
  From Workspace2 : FromWorkspace  VariableName=pitchrate_error  SampleTime=Tq  Interpolate=off  OutputAfterFinalValue=Holding final value
  pitchrate_error : Outport
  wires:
  From Workspace2/1 -> pitchrate_error/1

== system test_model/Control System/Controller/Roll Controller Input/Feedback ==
  roll_error_model : Inport
  roll_error : Outport
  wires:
  roll_error_model/1 -> roll_error/1

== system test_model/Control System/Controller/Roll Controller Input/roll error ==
  From Workspace4 : FromWorkspace  VariableName=roll_error  SampleTime=Tq  Interpolate=off  OutputAfterFinalValue=Holding final value
  roll_error : Outport
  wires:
  From Workspace4/1 -> roll_error/1

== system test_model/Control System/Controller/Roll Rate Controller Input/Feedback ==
  rollrate_error_model : Inport
  rollrate_error : Outport
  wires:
  rollrate_error_model/1 -> rollrate_error/1

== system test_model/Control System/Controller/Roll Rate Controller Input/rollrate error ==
  From Workspace5 : FromWorkspace  VariableName=rollrate_error  SampleTime=Tq  Interpolate=off  OutputAfterFinalValue=Holding final value
  rollrate_error : Outport
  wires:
  From Workspace5/1 -> rollrate_error/1

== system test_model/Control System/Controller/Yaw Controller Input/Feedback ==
  yaw_error_model : Inport
  yaw_error : Outport
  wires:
  yaw_error_model/1 -> yaw_error/1

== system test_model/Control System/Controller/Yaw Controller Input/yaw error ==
  From Workspace7 : FromWorkspace  VariableName=yaw_error  SampleTime=Tc  Interpolate=off  OutputAfterFinalValue=Holding final value
  yaw_error : Outport
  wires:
  From Workspace7/1 -> yaw_error/1

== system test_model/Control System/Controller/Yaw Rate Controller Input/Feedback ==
  yawrate_error_model : Inport
  yawrate_error : Outport
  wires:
  yawrate_error_model/1 -> yawrate_error/1

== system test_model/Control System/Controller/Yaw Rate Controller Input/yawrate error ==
  From Workspace8 : FromWorkspace  VariableName=yawrate_error  SampleTime=Tq  Interpolate=off  OutputAfterFinalValue=Holding final value
  yawrate_error : Outport
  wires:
  From Workspace8/1 -> yawrate_error/1

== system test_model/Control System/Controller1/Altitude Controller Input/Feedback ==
  z_error_model : Inport
  z_error : Outport
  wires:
  z_error_model/1 -> z_error/1

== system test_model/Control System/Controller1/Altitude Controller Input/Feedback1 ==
  z_position_model : Inport
  z_position : Outport
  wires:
  z_position_model/1 -> z_position/1

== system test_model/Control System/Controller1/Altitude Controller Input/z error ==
  From Workspace1 : FromWorkspace  VariableName=z_position  SampleTime=Tc  Interpolate=off  OutputAfterFinalValue=Holding final value
  From Workspace6 : FromWorkspace  VariableName=z_error  SampleTime=Tc  Interpolate=off  OutputAfterFinalValue=Holding final value
  z_error : Outport
  z_position : Outport  Port=2
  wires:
  From Workspace6/1 -> z_error/1
  From Workspace1/1 -> z_position/1

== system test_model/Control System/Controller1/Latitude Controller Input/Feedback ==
  x_error_model : Inport
  x_error : Outport
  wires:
  x_error_model/1 -> x_error/1

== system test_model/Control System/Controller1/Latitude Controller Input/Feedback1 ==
  x_position_model : Inport
  x_position : Outport
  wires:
  x_position_model/1 -> x_position/1

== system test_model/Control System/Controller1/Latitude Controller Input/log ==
  From Workspace : FromWorkspace  VariableName=x_error  SampleTime=Tc  Interpolate=off  OutputAfterFinalValue=Holding final value
  From Workspace1 : FromWorkspace  VariableName=x_position  SampleTime=Tc  Interpolate=off  OutputAfterFinalValue=Holding final value
  x_error : Outport
  x_position : Outport  Port=2
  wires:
  From Workspace/1 -> x_error/1
  From Workspace1/1 -> x_position/1

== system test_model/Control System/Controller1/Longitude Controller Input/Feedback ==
  y_error_model : Inport
  y_error : Outport
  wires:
  y_error_model/1 -> y_error/1

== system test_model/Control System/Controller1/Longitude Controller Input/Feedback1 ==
  y_position_model : Inport
  y_position : Outport
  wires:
  y_position_model/1 -> y_position/1

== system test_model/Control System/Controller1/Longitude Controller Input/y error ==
  From Workspace1 : FromWorkspace  VariableName=y_position  SampleTime=Tc  Interpolate=off  OutputAfterFinalValue=Holding final value
  From Workspace3 : FromWorkspace  VariableName=y_error  SampleTime=Tc  Interpolate=off  OutputAfterFinalValue=Holding final value
  y_error : Outport
  y_position : Outport  Port=2
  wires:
  From Workspace3/1 -> y_error/1
  From Workspace1/1 -> y_position/1

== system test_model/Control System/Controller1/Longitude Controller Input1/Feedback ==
  y_vel_error_model : Inport
  y_vel_error : Outport
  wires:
  y_vel_error_model/1 -> y_vel_error/1

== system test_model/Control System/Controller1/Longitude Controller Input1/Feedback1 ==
  y_vel_model : Inport
  y_vel : Outport
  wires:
  y_vel_model/1 -> y_vel/1

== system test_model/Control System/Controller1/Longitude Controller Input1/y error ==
  From Workspace1 : FromWorkspace  VariableName=y_vel  SampleTime=Tc  Interpolate=off  OutputAfterFinalValue=Holding final value
  From Workspace3 : FromWorkspace  VariableName=y_vel_error  SampleTime=Tc  Interpolate=off  OutputAfterFinalValue=Holding final value
  y_vel_error : Outport
  y_vel : Outport  Port=2
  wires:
  From Workspace3/1 -> y_vel_error/1
  From Workspace1/1 -> y_vel/1

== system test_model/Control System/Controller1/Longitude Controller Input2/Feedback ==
  x_vel_error_model : Inport
  x_vel_error : Outport
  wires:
  x_vel_error_model/1 -> x_vel_error/1

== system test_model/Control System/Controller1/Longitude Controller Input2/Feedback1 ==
  x_vel_model : Inport
  x_vel : Outport
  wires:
  x_vel_model/1 -> x_vel/1

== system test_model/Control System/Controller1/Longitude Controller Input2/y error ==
  From Workspace1 : FromWorkspace  VariableName=x_vel  SampleTime=Tc  Interpolate=off  OutputAfterFinalValue=Holding final value
  From Workspace3 : FromWorkspace  VariableName=x_vel_error  SampleTime=Tc  Interpolate=off  OutputAfterFinalValue=Holding final value
  x_vel_error : Outport
  x_vel : Outport  Port=2
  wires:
  From Workspace3/1 -> x_vel_error/1
  From Workspace1/1 -> x_vel/1

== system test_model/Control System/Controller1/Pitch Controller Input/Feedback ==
  pitch_error_model : Inport
  pitch_error : Outport
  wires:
  pitch_error_model/1 -> pitch_error/1

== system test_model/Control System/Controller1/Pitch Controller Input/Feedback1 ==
  pitch_angle_model : Inport
  pitch_angle : Outport
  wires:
  pitch_angle_model/1 -> pitch_angle/1

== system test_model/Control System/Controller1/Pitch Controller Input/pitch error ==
  From Workspace : FromWorkspace  VariableName=pitch_error  SampleTime=Tq  Interpolate=off  OutputAfterFinalValue=Holding final value
  From Workspace1 : FromWorkspace  VariableName=pitch_angle  SampleTime=Tq  Interpolate=off  OutputAfterFinalValue=Holding final value
  pitch_error : Outport
  pitch_angle : Outport  Port=2
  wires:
  From Workspace/1 -> pitch_error/1
  From Workspace1/1 -> pitch_angle/1

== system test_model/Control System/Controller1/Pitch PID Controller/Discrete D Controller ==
  pitch_angle : Inport
  Discrete Derivative : simulink/Discrete/Discrete Derivative  gainval=Kd  ICPrevScaledInput=0.0  OutMin=[]  OutMax=[]  OutDataType=fixdt(1, 16)  OutScaling=2^-10  DoSatur=off
  Discrete Filter : DiscreteFilter  Numerator=[0 a]  Denominator=[1-a]
  Sum : Sum  Inputs=|++
  output : Outport
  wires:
  Discrete Derivative/1 -> Sum/1
  Discrete Filter/1 -> Sum/2
  Sum/1 -> Discrete Filter/1, output/1
  pitch_angle/1 -> Discrete Derivative/1

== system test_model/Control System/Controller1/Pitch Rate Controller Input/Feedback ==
  pitchrate_error_model : Inport
  pitchrate_error : Outport
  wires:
  pitchrate_error_model/1 -> pitchrate_error/1

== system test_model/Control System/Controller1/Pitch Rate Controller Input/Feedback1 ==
  pitchrate_model : Inport
  pitchrate : Outport
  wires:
  pitchrate_model/1 -> pitchrate/1

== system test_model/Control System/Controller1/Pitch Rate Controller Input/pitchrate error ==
  From Workspace1 : FromWorkspace  VariableName=pitchrate  SampleTime=Tq  Interpolate=off  OutputAfterFinalValue=Holding final value
  From Workspace2 : FromWorkspace  VariableName=pitchrate_error  SampleTime=Tq  Interpolate=off  OutputAfterFinalValue=Holding final value
  pitchrate_error : Outport
  pitchrate : Outport  Port=2
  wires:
  From Workspace2/1 -> pitchrate_error/1
  From Workspace1/1 -> pitchrate/1
